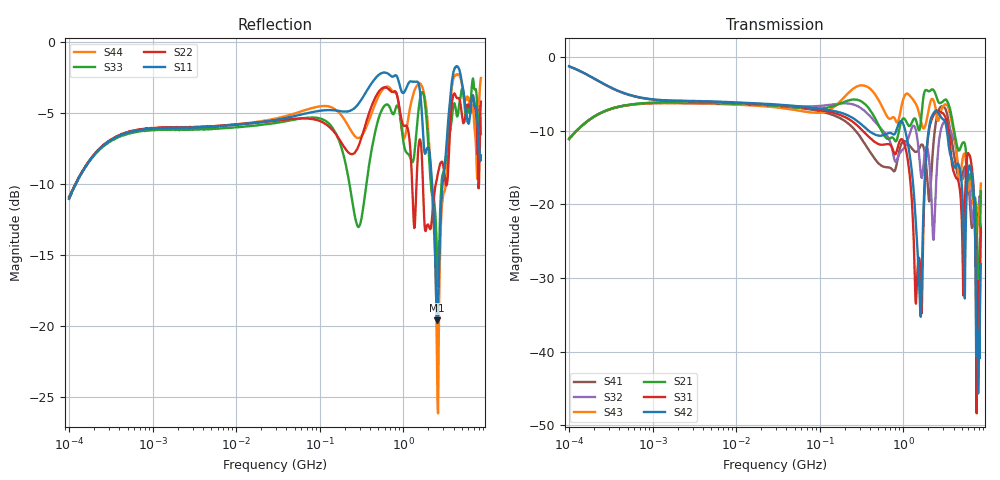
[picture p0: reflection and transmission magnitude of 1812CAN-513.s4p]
# Hz S dB R 50
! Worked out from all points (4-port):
!   801 points, 100 kHz to 8.5 GHz, reference 50 ohm
!   strongest paths, dB at 100 kHz, 1.721 MHz, 29.51 MHz, 502.3 MHz, 8.5 GHz:
!     S42: -1.3, -5.9, -6.4, -10.7, -28.2
!     S31: -1.3, -6.0, -6.5, -11.8, -23.3
!     S21: -11.1, -6.2, -6.6, -9.2, -18.3
!     S43: -11.1, -6.3, -6.8, -5.8, -17.2
!     S32: -11.1, -6.3, -6.6, -9.3, -20.3
!     S41: -11.2, -6.2, -6.6, -14.4, -23.7
!   lowest |S11| = -19.6 dB at 2.532 GHz (marker M1), VSWR 1.23, Z = 55.1 - j9.78 ohm
!   |S11| at or under -10 dB: start of sweep to 120.5 kHz; 2.22 GHz to 2.96 GHz (740.1 MHz wide, 28.6 % of centre)
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100000  -11.08 53.8  -11.17 55.2  -1.30 -15.2  -11.15 -125.7
        -11.15 55.0  -11.05 53.3  -11.12 -125.1  -1.29 -15.3
        -1.30 -15.1  -11.12 -125.4  -10.94 54.5  -11.15 54.4
        -11.18 -125.3  -1.26 -15.3  -11.09 54.2  -10.95 54.5
9.499517e8  -3.48 18.6  -8.72 13.2  -11.17 64.2  -11.79 -131.9
            -8.73 13.2  -5.47 10.2  -12.77 -133.8  -8.73 59.6
            -11.16 64.1  -12.77 -133.9  -5.96 19.2  -6.78 9.3
            -11.80 -132.0  -8.73 59.6  -6.78 9.3  -5.95 17.9
1.583696e9  -3.47 13.0  -9.73 23.5  -28.05 95.1  -12.23 115.2
            -9.72 23.5  -6.89 44.6  -14.60 11.7  -33.37 -46.7
            -28.02 95.9  -14.59 11.6  -4.05 62.8  -8.13 -23.2
            -12.24 115.2  -33.45 -46.5  -8.13 -23.2  -2.94 38.4
2.531803e9  -19.62 -57.3  -5.64 -13.9  -7.27 53.9  -8.10 83.7
            -5.63 -13.9  -9.67 124.2  -15.03 55.7  -7.32 37.6
            -7.29 53.8  -15.00 55.4  -14.94 85.2  -8.20 -22.3
            -8.10 83.6  -7.32 37.7  -8.19 -22.3  -21.92 -8.0
5.161627e9  -3.25 -100.1  -11.60 -22.7  -28.81 -37.8  -15.84 -38.0
            -11.63 -22.9  -5.58 -93.0  -16.43 -74.7  -19.83 -68.8
            -28.59 -37.9  -16.53 -75.5  -3.39 -87.8  -13.68 -14.7
            -15.84 -38.2  -19.77 -68.6  -13.69 -14.4  -3.42 -99.6
6.842542e9  -3.79 10.4  -18.70 -31.1  -16.66 -64.4  -22.37 94.7
            -18.71 -30.9  -3.79 7.1  -22.53 116.9  -17.28 -79.7
            -16.63 -64.7  -22.44 116.5  -2.60 15.9  -19.68 -18.7
            -22.43 95.0  -17.25 -79.4  -19.68 -18.3  -4.93 -5.4
8.5e9  -8.01 129.8  -18.30 78.8  -23.34 73.6  -23.74 18.4
       -18.25 78.6  -4.24 128.2  -20.26 13.5  -28.13 38.8
       -23.30 73.3  -20.27 13.0  -6.52 120.2  -17.15 45.0
       -23.73 18.2  -28.17 38.5  -17.19 45.4  -2.57 128.4
